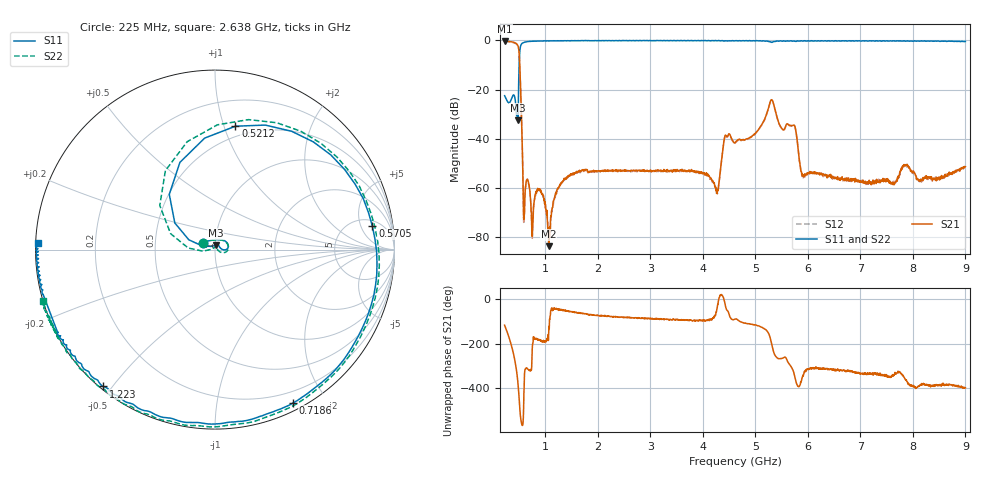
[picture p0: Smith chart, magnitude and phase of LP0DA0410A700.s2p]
!Agilent Technologies,E8358A,US41080443,A.07.50.56
!Agilent E8358A: A.07.50.56
!Date: Wednesday, August 31, 2016 09:02:10
!Correction: S11(Full 2 Port(1,2))
!S21(Full 2 Port(1,2))
!S12(Full 2 Port(1,2))
!S22(Full 2 Port(1,2))
!S2P File: Measurements: S11, S21, S12, S22:
# Hz S  dB  R 50
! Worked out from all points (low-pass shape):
!   1601 points, 225 MHz to 9 GHz, reference 50 ohm
!   highest |S21| = -0.23 dB at 225 MHz (marker M1); lowest = -83.7 dB at 1.064 GHz (marker M2)
!   |S21| within 3 dB of the highest: start of sweep to 492 MHz
!   lowest |S11| = -32.4 dB at 477.3 MHz (marker M3), VSWR 1.05, Z = 50.3 + j2.38 ohm
!   |S11| at or under -10 dB: start of sweep to 501.5 MHz
!   |S22| runs from -38.0 to 0.1 dB; largest |S21 - S12| = 0.022
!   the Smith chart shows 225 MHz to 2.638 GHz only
!   S11 on the Smith chart (normalised r, x): 225 MHz: 0.87, +0.06; 521.2 MHz: 0.41, +1.09; 570.5 MHz: 7, +8; 718.6 MHz: 0.08, -1.63; 1.223 GHz: 0.01, -0.47; 2.638 GHz: 0.01, +0.02
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2.25e8  -22.49 152.6  -0.23 -117.9  -0.41 -117.6  -22.31 152.0
3.237188e8  -25.17 83.5  -0.43 176.3  -0.62 176.6  -25.14 81.2
3.950156e8  -22.17 23.7  -0.75 112.7  -0.93 112.9  -22.28 17.4
4.772812e8  -32.42 81.8  -2.07 -12.8  -2.25 -12.6  -36.35 81.9
5.211562e8  -3.14 80.6  -14.24 -154.2  -14.41 -153.9  -3.16 88.9
5.705156e8  -1.04 8.4  -51.71 154.2  -51.96 155.5  -0.98 12.5
6.089062e8  -0.70 -19.3  -64.52 35.9  -65.74 39.2  -0.61 -16.4
7.185938e8  -0.37 -62.9  -64.78 37.3  -64.59 39.3  -0.25 -61.6
9.050625e8  -0.21 -99.3  -60.82 172.5  -60.47 171.9  -0.07 -99.1
1.064109e9  -0.21 -117.5  -83.66 -153.6  -80.06 -76.7  -0.07 -117.6
1.223156e9  -0.14 -129.2  -60.78 -46.9  -61.46 -42.9  0.00 -130.1
1.689328e9  -0.06 -150.1  -52.87 -63.4  -53.34 -64.0  0.03 -153.7
2.638125e9  -0.11 178.0  -52.77 -85.0  -53.13 -84.0  0.00 -163.2
3.153656e9  -0.12 172.0  -52.69 -89.5  -53.19 -90.9  0.00 -167.9
4.2615e9  -0.14 161.4  -61.04 -53.3  -59.71 -50.5  -0.01 -179.3
4.431516e9  -0.14 160.1  -38.52 -32.0  -38.74 -31.9  -0.04 178.5
4.6125e9  -0.15 158.8  -41.51 -90.2  -41.82 -89.2  -0.01 176.5
5.3145e9  -0.78 148.2  -24.12 153.6  -24.32 153.7  -0.63 163.1
5.906812e9  -0.26 138.6  -54.82 16.9  -55.38 18.8  -0.13 149.4
6.076828e9  -0.16 134.6  -53.75 51.3  -53.91 49.3  -0.09 143.8
7.541156e9  -0.27 108.7  -57.49 11.9  -56.89 10.9  -0.18 105.1
9e9  -0.41 78.6  -51.36 -39.1  -51.00 -38.1  -0.30 65.6
